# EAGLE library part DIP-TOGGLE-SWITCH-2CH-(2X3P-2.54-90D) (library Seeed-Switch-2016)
311030004
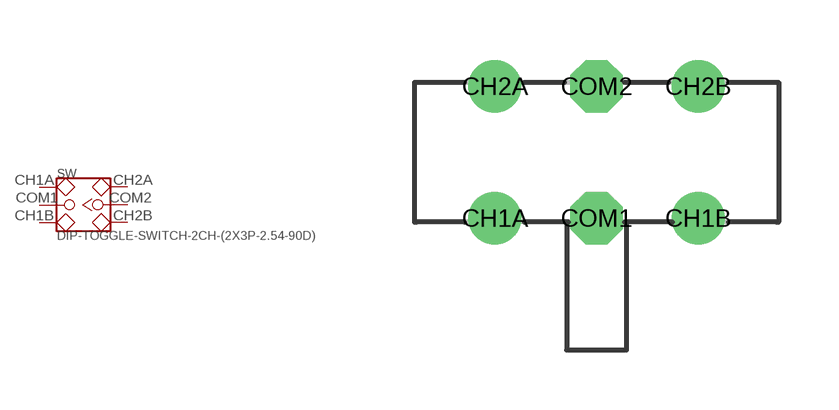
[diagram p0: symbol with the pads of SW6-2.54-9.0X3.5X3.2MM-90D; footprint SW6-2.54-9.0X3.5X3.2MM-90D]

Designator prefix SW

## DIP-TOGGLE-SWITCH-2CH-(2X3P-2.54-90D)'90D'  [SW6-2.54-9.0X3.5X3.2MM-90D]
CH1A  CH1A
CH1B  CH1B
CH2A  CH2A
CH2B  CH2B
COM1  COM1
COM2  COM2

## Footprint SW6-2.54-9.0X3.5X3.2MM-90D (pad centres in mm)
drill 0.813 pad 1.27: CH1A -2.54,-1.65; CH1B 2.54,-1.65; CH2A -2.54,1.65; CH2B 2.54,1.65
drill 0.813 pad 1.27 octagon: COM1 0,-1.65; COM2 0,1.65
